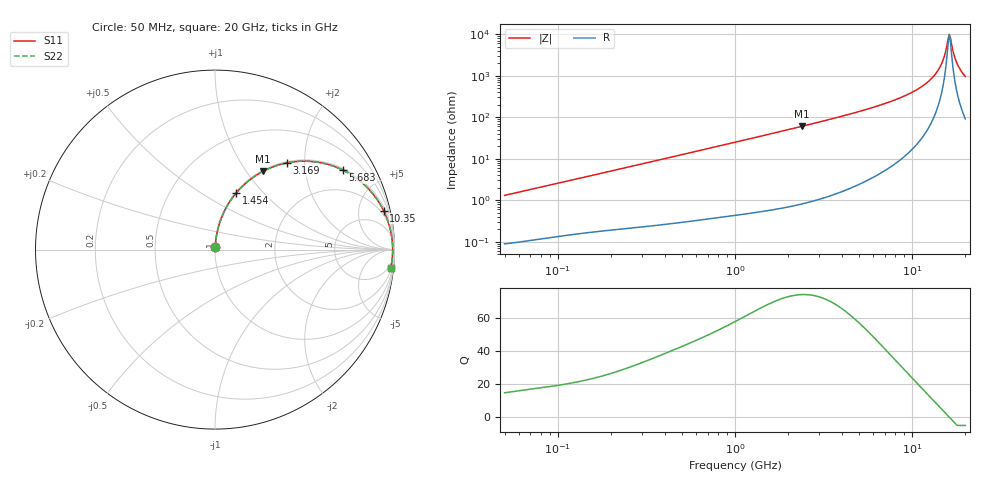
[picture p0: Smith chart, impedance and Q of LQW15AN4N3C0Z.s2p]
!Murata Part Number: LQW15AN4N3C0Z
!These Parameters are Measured in Series Mode Connection
!  o--[Z]--o
!Port1  Port2
!  o-------o
!Freq. Start=50[MHz] Stop=20[GHz], 401[Steps]
# Hz S RI R 50
!Freq.(Hz) S11(Real) S11(Imag) S21(Real) S21(Imag) S12(Real) S12(Imag) S22(Real) S22(Imag)
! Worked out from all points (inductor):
!   401 points, 50 MHz to 20 GHz, reference 50 ohm
!   read as one part in series: L = 4.13 nH near 51.52 MHz
!   highest Q = 74 at 2.384 GHz (marker M1), where L = 4.01 nH
!   self-resonance near 16.22 GHz
!   S11 on the Smith chart (normalised r, x): 50 MHz: 1.00, +0.03; 1.454 GHz: 1.01, +0.72; 3.169 GHz: 1.02, +1.62; 5.683 GHz: 1.06, +3.19; 10.35 GHz: 1.39, +8.56; 20 GHz: 3, -19
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5e7  0.00106 0.013  0.9989 -0.013  0.9989 -0.013  0.00106 0.013
1.364002e8  0.00279 0.0346  0.9972 -0.0346  0.9972 -0.0346  0.00279 0.0346
3.721004e8  0.011 0.0918  0.989 -0.0918  0.989 -0.0918  0.011 0.0918
1e9  0.0618 0.2322  0.9382 -0.2322  0.9382 -0.2322  0.0618 0.2322
1.454215e9  0.1196 0.3171  0.8804 -0.3171  0.8804 -0.3171  0.1196 0.3171
2.383959e9  0.2681 0.4362  0.7319 -0.4362  0.7319 -0.4362  0.2681 0.4362
2.728004e9  0.3261 0.462  0.6739 -0.462  0.6739 -0.462  0.3261 0.462
3.168813e9  0.3987 0.4827  0.6013 -0.4827  0.6013 -0.4827  0.3987 0.4827
5.683258e9  0.7142 0.4422  0.2858 -0.4422  0.2858 -0.4422  0.7142 0.4422
7.442007e9  0.8369 0.3566  0.1631 -0.3566  0.1631 -0.3566  0.8369 0.3566
1.034674e10  0.9395 0.2167  0.0605 -0.2167  0.0605 -0.2167  0.9395 0.2167
1.220001e10  0.9697 0.1391  0.0303 -0.1391  0.0303 -0.1391  0.9697 0.1391
1.375312e10  0.9831 0.0812  0.0169 -0.0812  0.0169 -0.0812  0.9831 0.0812
1.482269e10  0.9878 0.0447  0.0122 -0.0447  0.0122 -0.0447  0.9878 0.0447
1.527346e10  0.989 0.03  0.011 -0.03  0.011 -0.03  0.989 0.03
1.573793e10  0.9897 0.0154  0.0103 -0.0154  0.0103 -0.0154  0.9897 0.0154
1.621653e10  0.9899 0.000699  0.0101 -0.000699  0.0101 -0.000699  0.9899 0.000699
1.670968e10  0.9897 -0.014  0.0103 0.014  0.0103 0.014  0.9897 -0.014
1.747767e10  0.9886 -0.036  0.0114 0.036  0.0114 0.036  0.9886 -0.036
1.800918e10  0.9874 -0.0506  0.0126 0.0506  0.0126 0.0506  0.9874 -0.0506
1.912117e10  0.9835 -0.0799  0.0165 0.0799  0.0165 0.0799  0.9835 -0.0799
2e10  0.9795 -0.1017  0.0205 0.1017  0.0205 0.1017  0.9795 -0.1017
